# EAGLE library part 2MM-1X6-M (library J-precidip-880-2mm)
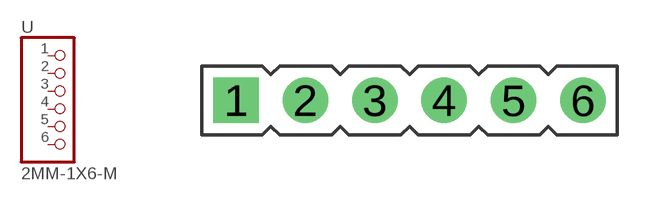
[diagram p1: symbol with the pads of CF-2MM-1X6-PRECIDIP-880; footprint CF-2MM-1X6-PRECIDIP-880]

Designator prefix -

## 2MM-1X6-M  [CF-2MM-1X6-PRECIDIP-880]
1  1  pas
2  2  pas
3  3  pas
4  4  pas
5  5  pas
6  6  pas

## Footprint CF-2MM-1X6-PRECIDIP-880 (pad centres in mm)
Pin Header, 1x6, 2.00mm, Through Hole Preci-Dip pn: 880-70-006-10-001101
drill 0.8 square: 1 0,0
drill 0.8: 2 2,0; 3 4,0; 4 6,0; 5 8,0; 6 10,0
